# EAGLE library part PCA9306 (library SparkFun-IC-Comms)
Bidirectional I2C level shifter Not compatible with all available part number pinout schemes- DOUBLE CHECK!!! Datasheet SparkFun Products SparkFun Inventor's Kit for RedBot (ROB-12649) SparkFun RedBot Basic Kit (ROB-13166) SparkFun Level Translator Breakout - PCA9306 (BOB-11955) SparkFun Block for Intel Edison - ADC (DEV-13770) SparkFun Block for Intel® Edison - Raspberry Pi B (DEV-13044) SparkFun RedBot Sensor - Accelerometer (SEN-12589)
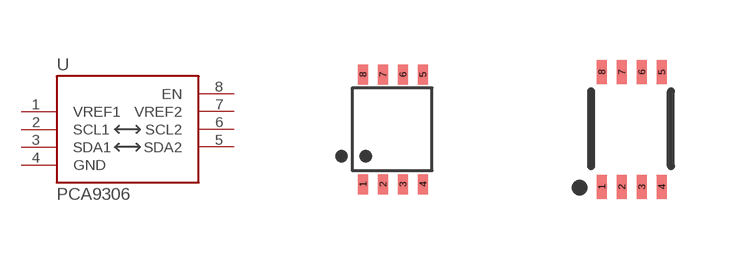
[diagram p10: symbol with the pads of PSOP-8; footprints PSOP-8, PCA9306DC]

Designator prefix U

## PCA9306 (PROD_ID: IC-10023; VALUE: PCA9306)  [PSOP-8]
1  VREF1
2  SCL1
3  SDA1
4  GND
5  SDA2
6  SCL2
7  VREF2
8  EN

## PCA9306PCA9306DC-1:1 (PROD_ID: IC-10023; VALUE: PCA9306)  [PCA9306DC]
Pads as for PSOP-8

## Footprint PSOP-8 (pad centres in mm)
PSOP-8 Specifications: Pin count:8 Example device(s): PCA9306
smd 0.25 x 0.5: 1 -0.73,-1.37; 2 -0.23,-1.37; 3 0.27,-1.37; 4 0.77,-1.37; 5 0.77,1.38; 6 0.27,1.38; 7 -0.23,1.38; 8 -0.73,1.38

## Footprint PCA9306DC (pad centres in mm)
PCA9306DC 1:1 package. Specifications: Pin count: 8 Example device(s): PCA9306
smd 0.25 x 0.602: 1 -0.73,-1.446; 2 -0.23,-1.446; 3 0.27,-1.446; 4 0.77,-1.446; 5 0.77,1.431; 6 0.27,1.431; 7 -0.23,1.431; 8 -0.73,1.431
